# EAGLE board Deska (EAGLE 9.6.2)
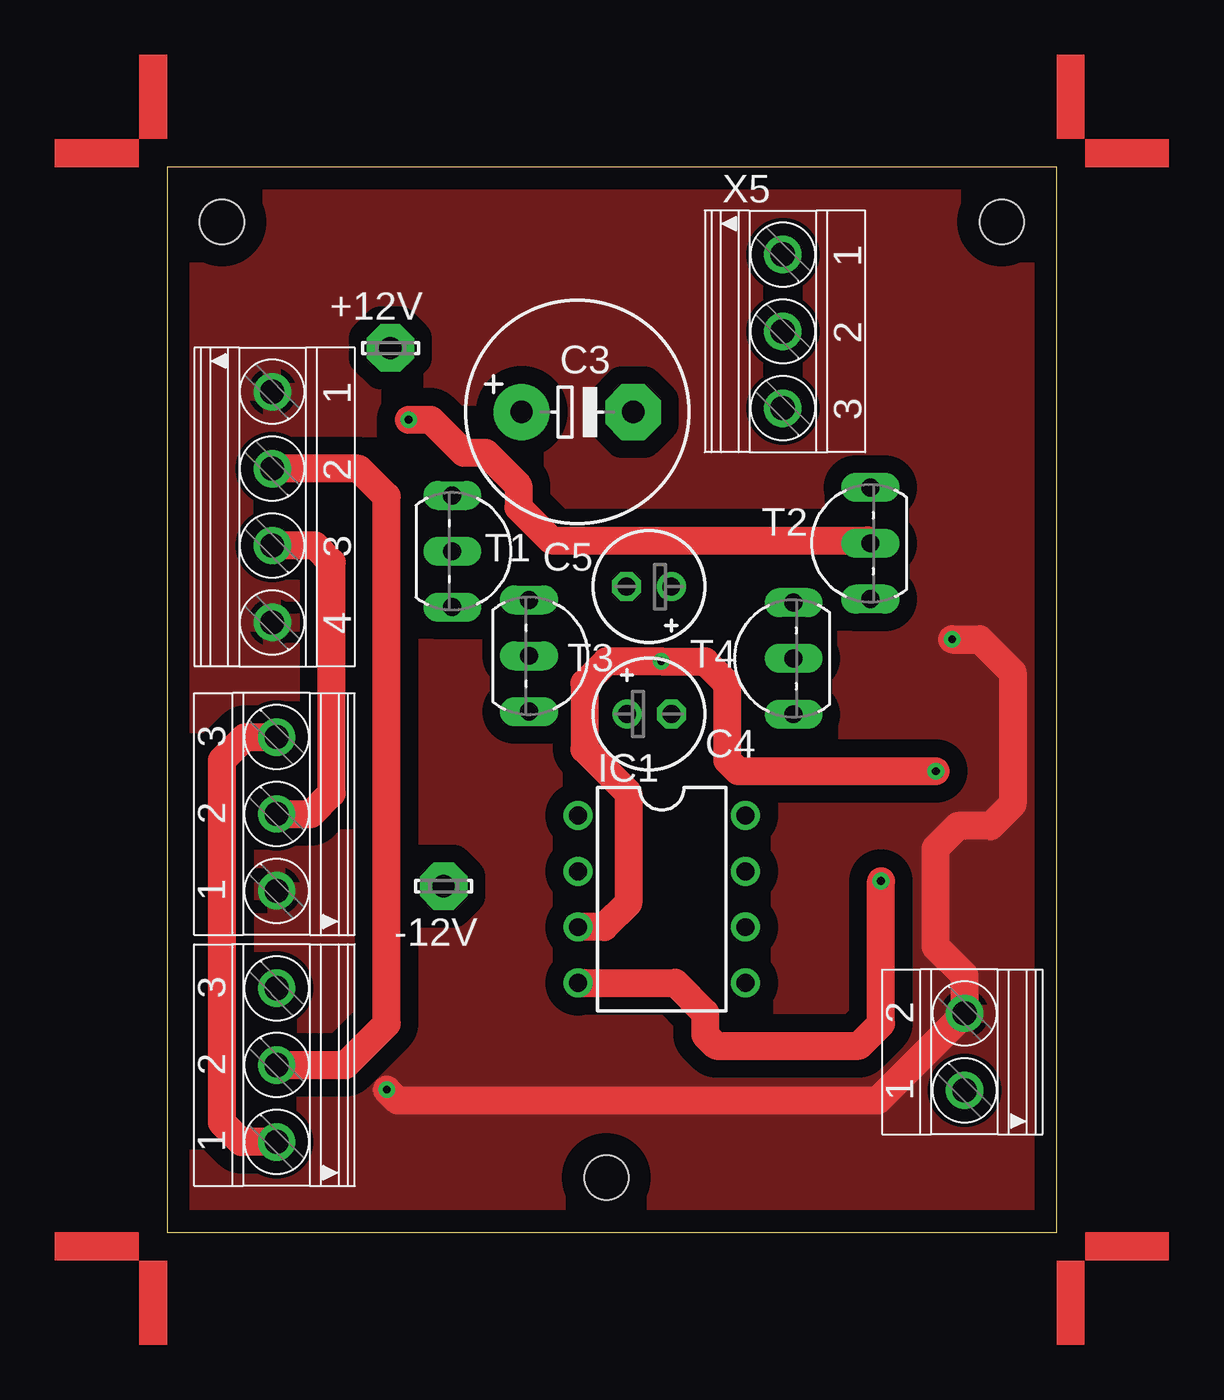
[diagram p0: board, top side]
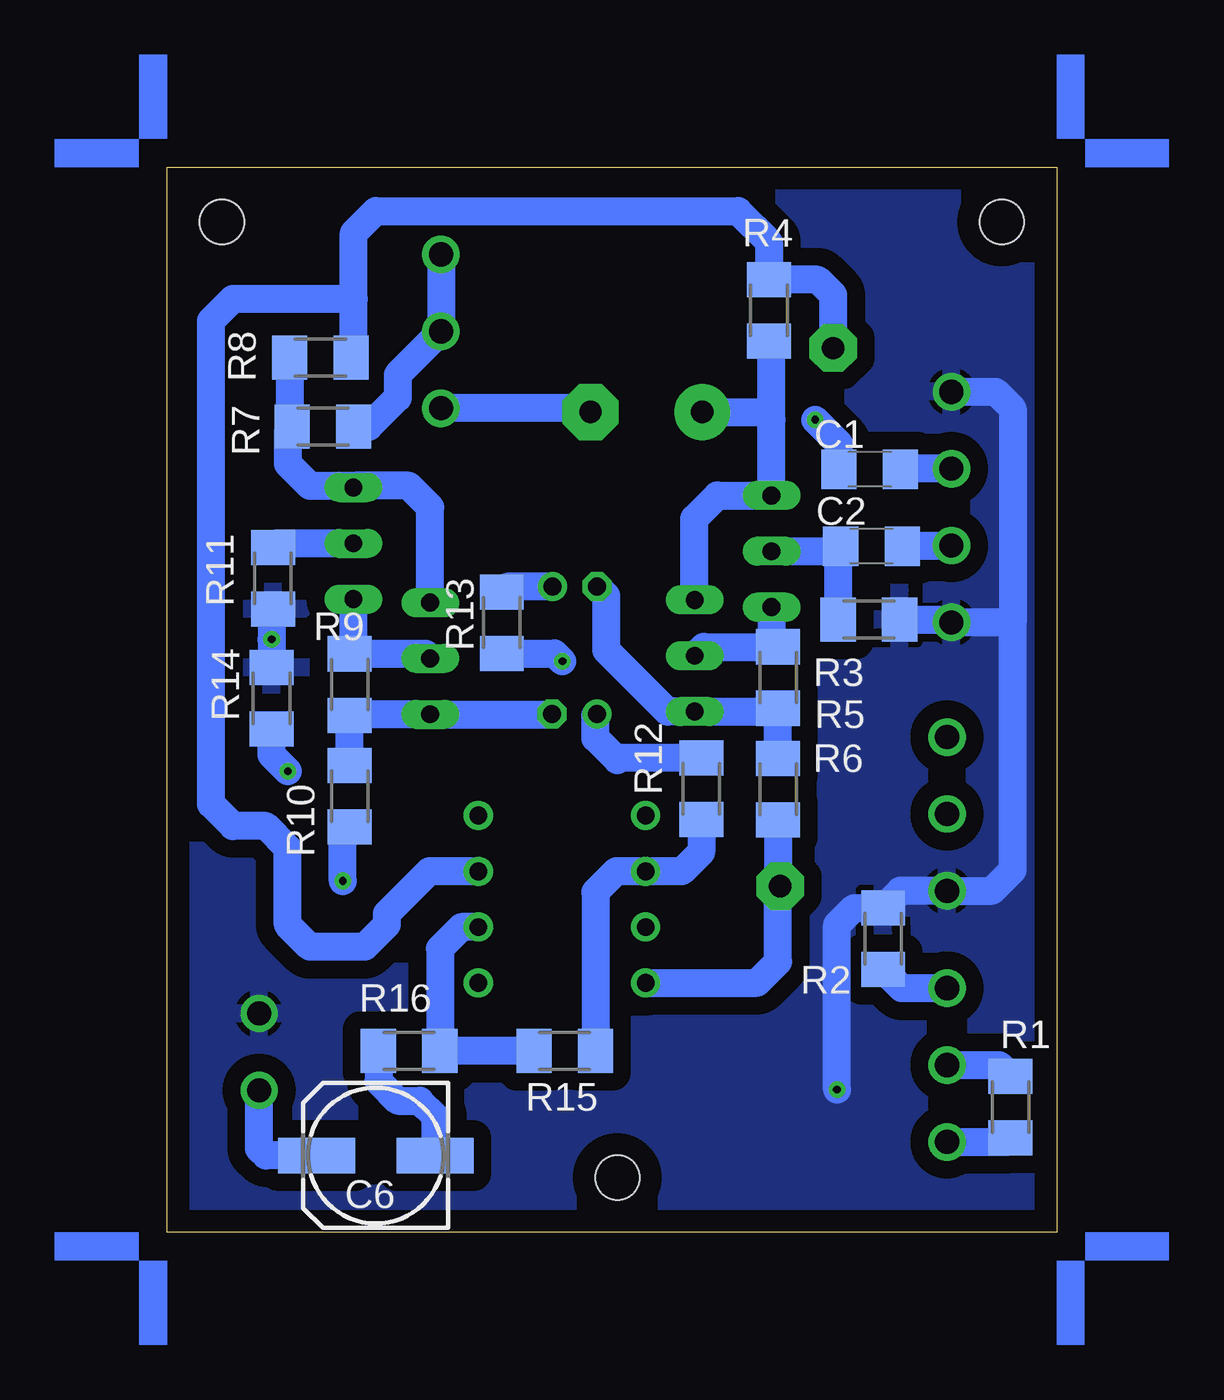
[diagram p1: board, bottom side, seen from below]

Size 40.5 x 48.5 mm. Coordinates in mm from the lower left corner, seen from the top.
Outline: 0,0 40.5,0 40.5,48.5 0,48.5 0,0
Copper layers (1*16): Top 0.035mm / dielectric 1.5mm / Bottom 0.035mm
Design rules "default": minimum track width 6mil, minimum drill 0.35mm, track to track 6mil, track to pad 6mil, pad to pad 6mil, via to via 6mil, smd to smd 6mil, copper to edge 40mil, drill to drill 6mil, minimum pad ring 10mil, minimum via ring 8mil, stop-mask expansion 4mil, vias tented up to drill 0mil, thermal gap 10mil
Holes 2 mm at 2.5,46 38,46 20,2.5

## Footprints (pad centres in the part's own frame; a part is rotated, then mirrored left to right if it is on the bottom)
LSP10 = drill 1.016 pad 2.159 octagon: MP 0,0
C1206 = smd 1.6 x 1.8: 1 -1.4,0; 2 1.4,0
E5-10,5 = drill 1.016 pad 2.54: + -2.54,0 | drill 1.016 pad 2.54 octagon: - 2.54,0
E2-5 = drill 0.813 pad 1.27: + -1.016,0 | drill 0.813 pad 1.27 octagon: - 1.016,0
153CLV-0605 = smd 3.5 x 1.6: + 2.7,0; - -2.7,0
DIL08 = drill 0.813 pad 1.27: 1 -3.81,-3.81; 2 -1.27,-3.81; 3 1.27,-3.81; 4 3.81,-3.81; 5 3.81,3.81; 6 1.27,3.81; 7 -1.27,3.81; 8 -3.81,3.81
M1206 = smd 1.6 x 2: 1 -1.4,0; 2 1.4,0
TO92-EBC = drill 0.813 long: B 0,-1.27; C 2.54,-1.27; E -2.54,-1.27
TO92-CBE = drill 0.813 long: B 0,0; C -2.54,0; E 2.54,0
1751251 = drill 1.1 pad 1.7: 1 -3.5,-0.1; 2 0,-0.1; 3 3.5,-0.1
1751264 = drill 1.1 pad 1.7: 1 -5.25,-0.1; 2 -1.75,-0.1; 3 1.75,-0.1; 4 5.25,-0.1
1751248 = drill 1.1 pad 1.7: 1 -1.75,-0.1; 2 1.75,-0.1

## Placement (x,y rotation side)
+12V  LSP10  [LSP10]  10.17,40.26 0 top
-12V  LSP10  [LSP10]  12.59,15.76 0 top
C1  [C1206]  8.51,34.74 180 bottom
C2  [C1206]  8.43,31.24 180 bottom
C3  [E5-10,5]  18.68,37.35 0 top
C4  [E2-5]  21.95,23.6 0 top
C5  [E2-5]  21.94,29.4 180 top
C6  [153CLV-0605]  31,3.5 180 bottom
IC1  TL071P  [DIL08]  22.52,15.17 270 top
R1  [M1206]  2.1,5.71 90 bottom
R2  [M1206]  7.9,13.37 270 bottom
R3  [M1206]  8.55,27.9 180 bottom
R4  [M1206]  13.1,41.97 90 bottom
R5  [M1206]  12.68,25.26 90 bottom
R6  [M1206]  12.68,20.18 90 bottom
R7  [M1206]  33.4,36.68 0 bottom
R8  [M1206]  33.52,39.82 180 bottom
R9  [M1206]  32.18,24.94 90 bottom
R10  [M1206]  32.18,19.86 90 bottom
R11  [M1206]  35.68,29.78 90 bottom
R12  [M1206]  16.18,20.2 90 bottom
R13  [M1206]  25.26,27.76 90 bottom
R14  [M1206]  35.74,24.32 270 bottom
R15  [M1206]  22.4,8.26 0 bottom
R16  [M1206]  29.48,8.26 0 bottom
T1  [TO92-EBC]  14.25,31.01 270 top
T2  [TO92-EBC]  30.75,31.37 90 top
T3  [TO92-CBE]  16.48,26.25 270 top
T4  [TO92-CBE]  28.52,26.13 90 top
U$1  [ANGLE-SW1-16]  40.5,48.5 0 top
U$2  [ANGLE-SW1-16]  0,48.5 90 top
U$3  [ANGLE-SW1-16]  0,0 180 top
U$4  [ANGLE-SW1-16]  40.5,0 270 top
X1  [1751251]  4.89,7.62 90 top
X2  [1751251]  4.89,19.05 90 top
X3  [1751264]  4.89,33.02 270 top
X4  [1751248]  36.21,8.22 90 top
X5  [1751251]  28.13,41.02 270 top

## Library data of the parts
+12V -12V = solpad
C1-C6 = rcl; SPICEPREFIX: C
IC1 = linear
R1-R16 = rcl; SPICEPREFIX: R
T1-T4 = transistor
U$1-U$4 = marks
X1 X2 X4 X5 = con-phoenix-350; OC_FARNELL: unknown; OC_NEWARK: unknown
X3 = con-phoenix-350; MPN: 1751264; OC_FARNELL: unknown; OC_NEWARK: 10R0934

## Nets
+12V: +12V.MP IC1.7 R4.2 R8.1
-12V: -12V.MP IC1.4 R6.1 R10.1
GND: R2.1 R3.1 R11.1 R14.1 X2.1 X3.1 X3.4 X4.2
N$1: R1.1 X1.1 X2.3
N$2: C3.- X5.3
N$3: C2.1 X2.2 X3.3
N$4: R2.2 X1.3
N$5: C3.+ R4.1 T1.E T3.C
N$6: C2.2 R3.2 T1.B
N$7: R7.1 R8.2 T2.C T4.E
N$8: C1.1 R1.2 X1.2 X3.2
N$9: R7.2 X5.1 X5.2
N$10: C5.- R5.1 R6.2 T3.E
N$11: C4.- R9.1 R10.2 T4.C
N$12: R5.2 T1.C T3.B
N$13: R9.2 T2.E T4.B
N$14: C1.2 R11.2 T2.B
N$15: C4.+ R12.2
N$16: C5.+ R13.2
N$17: IC1.2 R12.1 R15.2
N$18: IC1.3 R13.1 R14.2
N$19: C6.- R16.1
N$20: IC1.6 R15.1 R16.2
N$23: C6.+ X4.1

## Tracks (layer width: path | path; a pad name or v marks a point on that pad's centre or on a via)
+12V
  Bottom 1.27: R8.1 32,39.94 32,42.5 | 32,42.5 32,45.5 31,46.5 14.5,46.5 13.1,45.1 R4.2 10.87,43.37 10.17,42.67 +12V.MP | IC1.7 28.56,16.44 30.5,14.5 30.5,14 31.5,13 34,13 35,14 35,17.5 36,18.5 37.5,18.5 38.5,19.5 38.5,41.5 37.5,42.5 32,42.5
-12V  (via drill 0.35)
  Top 1.27: IC1.4 23.14,11.36 24.5,10 24.5,9 25,8.5 31.5,8.5 32.5,9.5 v32.5,16
  Bottom 1.27: R10.1 32.5,18.14 v32.5,16 | R6.1 12.68,15.85 | 12.68,15.85 -12V.MP | IC1.4 13.64,11.36 12.68,12.32 12.68,15.85
GND  (via drill 0.35)
  Top 1.27: v35.74,27 37,27 38.5,25.5 38.5,19.5 37.5,18.5 36,18.5 35,17.5 35,13 36.31,11.69 X4.2 32.34,6 10.5,6 v10,6.5
  Bottom 1.27: 2,27.77 2,16.5 2.95,15.55 X2.1 7.12,15.55 R2.1 9.23,14.77 10,14 v10,6.5 | 2,27.77 X3.4 4.92,27.9 R3.1 | X3.1 2.77,38.27 2,37.5 2,27.77 | R11.1 35.74,28.32 v35.74,27 R14.1
  pour Top (isolate 0.813): 0,0 40.5,0 40.5,48.5 0,48.5
  pour Bottom (isolate 0.813): 0,0 40.5,0 40.5,48.5 0,48.5
N$1
  Top 1.27: X1.1 3.38,4.12 2.5,5 2.5,21.5 3.55,22.55 X2.3
  Bottom 1.27: X1.1 2.29,4.12 R1.1
N$2
  Bottom 1.27: C3.- 21.39,37.52 X5.3
N$3
  Top 1.27: X2.2 6.55,19.05 7.5,20 7.5,30.5 6.73,31.27 X3.3
  Bottom 1.27: X3.3 4.82,31.24 C2.1
N$4
  Bottom 1.27: X1.3 7.05,11.12 R2.2
N$5
  Bottom 1.27: 12.98,37 T1.E 15.45,33.55 16.5,32.5 16.48,32.48 T3.C | 12.98,37 12.98,40.45 R4.1 | C3.+ 13.33,37.35 12.98,37
N$6
  Bottom 1.27: R3.2 9.95,31.12 C2.2 10.06,31.01 T1.B
N$7
  Bottom 1.27: T4.E 28.52,33.02 29.5,34 31.93,34 | 31.93,34 T2.C | 31.93,34 34,34 35,35 35,36.48 R7.1 34.92,36.8 R8.2
N$8
  Top 1.27: X1.2 8.12,7.62 10,9.5 10,33.5 8.73,34.77 X3.2
  Bottom 1.27: X1.2 2.61,7.62 R1.2 | X3.2 7.08,34.77 C1.1
N$9
  Bottom 1.27: X5.1 X5.2 30,39.05 30,38 31.32,36.68 R7.2
N$10
  Bottom 1.27: 12.83,23.71 T3.E 17.71,23.71 20.5,26.5 20.5,28.98 C5.- | 12.83,23.71 R5.1 | R6.2 12.68,23.56 12.83,23.71
N$11
  Bottom 1.27: R10.2 R9.1 32.13,23.59 T4.C C4.-
N$12
  Bottom 1.27: T1.C 12.98,26.96 R5.2 16.07,26.66 T3.B
N$13
  Bottom 1.27: T4.B 28.73,26.34 R9.2 32.02,26.5 T2.E
N$14  (via drill 0.35)
  Top 1.27: v11,37 12,37 13.5,35.5 14.5,35.5 16,34 16,33 17.5,31.5 31.89,31.5 T2.B
  Bottom 1.27: T2.B 35.49,31.37 R11.2 | C1.2 9.91,35.91 v11,37
N$15
  Bottom 1.27: R12.2 19.9,21.6 20,21.5 21,22.5 21,23.53 C4.+
N$16
  Bottom 1.27: C5.+ 25.02,29.4 R13.2
N$17
  Bottom 1.27: R12.1 16.18,17.32 17.06,16.44 IC1.2 20.06,16.44 21,15.5 R15.2
N$18  (via drill 0.35)
  Top 1.27: IC1.3 19.9,13.9 21,15 21,20 19,22 19,25 20,26 v22.5,26 24.5,26 25.5,25 25.5,21.5 26,21 v35,21
  Bottom 1.27: R13.1 22.86,26.36 v22.5,26 | v35,21 35.74,21.74 R14.2
N$19
  Bottom 1.27: R16.1 30.88,6.88 30,6 29,6 28.3,5.3 C6.-
N$20
  Bottom 1.27: R15.1 R16.2 28.08,12.92 27.1,13.9 IC1.6
N$23
  Bottom 1.27: C6.+ 36,3.5 36.31,3.81 X4.1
